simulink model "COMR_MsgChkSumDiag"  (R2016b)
settings: Solver=FixedStepDiscrete  StartTime=0.0  StopTime=10.0  FixedStep=0.01  RelTol=1e-3  EnableMultiTasking=on
undefined symbols (not defined in the file or in its folder): bin2dec, COMR_cntABM050ChkSumDiag_CW, COMR_cntOBCChkSumDiag_CW, COMR_cntVcu2A3ChkSumDiag_CW
libraries: simulink x34

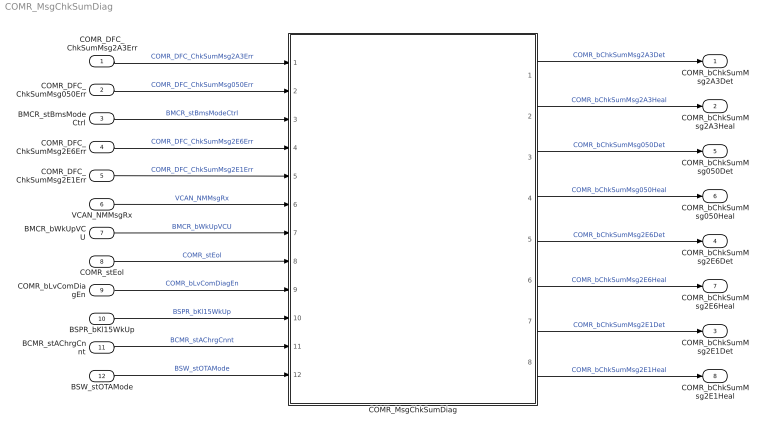
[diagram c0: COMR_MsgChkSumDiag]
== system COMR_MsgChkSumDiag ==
  COMR_DFC_ChkSumMsg2A3Err : Inport  OutDataTypeStr=boolean
  COMR_DFC_ChkSumMsg050Err : Inport  Port=2  OutDataTypeStr=boolean
  BMCR_stBmsModeCtrl : Inport  Port=3
  COMR_DFC_ChkSumMsg2E6Err : Inport  Port=4  OutDataTypeStr=boolean
  COMR_DFC_ChkSumMsg2E1Err : Inport  Port=5  OutDataTypeStr=boolean
  VCAN_NMMsgRx : Inport  Port=6  OutDataTypeStr=boolean
  BMCR_bWkUpVCU : Inport  Port=7  OutDataTypeStr=boolean
  COMR_stEol : Inport  Port=8  OutDataTypeStr=boolean
  COMR_bLvComDiagEn : Inport  Port=9  OutDataTypeStr=boolean
  BSPR_bKl15WkUp : Inport  Port=10
  BCMR_stAChrgCnnt : Inport  Port=11
  BSW_stOTAMode : Inport  Port=12  OutDataTypeStr=boolean
  COMR_MsgChkSumDiag : Subsystem
  COMR_bChkSumMsg2A3Det : Outport
  COMR_bChkSumMsg2A3Heal : Outport  Port=2
  COMR_bChkSumMsg2E1Det : Outport  Port=3
  COMR_bChkSumMsg2E6Det : Outport  Port=4
  COMR_bChkSumMsg050Det : Outport  Port=5
  COMR_bChkSumMsg050Heal : Outport  Port=6
  COMR_bChkSumMsg2E6Heal : Outport  Port=7
  COMR_bChkSumMsg2E1Heal : Outport  Port=8
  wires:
  COMR_DFC_ChkSumMsg2A3Err/1 -> COMR_MsgChkSumDiag/1(COMR_DFC_ChkSumMsg2A3Err)  "COMR_DFC_ChkSumMsg2A3Err"
  COMR_DFC_ChkSumMsg050Err/1 -> COMR_MsgChkSumDiag/2(COMR_DFC_ChkSumMsg050Err)  "COMR_DFC_ChkSumMsg050Err"
  COMR_DFC_ChkSumMsg2E6Err/1 -> COMR_MsgChkSumDiag/4(COMR_DFC_ChkSumMsg2E6Err)  "COMR_DFC_ChkSumMsg2E6Err"
  COMR_MsgChkSumDiag/1(COMR_bChkSumMsg2A3Det) -> COMR_bChkSumMsg2A3Det/1  "COMR_bChkSumMsg2A3Det"
  COMR_DFC_ChkSumMsg2E1Err/1 -> COMR_MsgChkSumDiag/5(COMR_DFC_ChkSumMsg2E1Err)  "COMR_DFC_ChkSumMsg2E1Err"
  COMR_MsgChkSumDiag/3(COMR_bChkSumMsg050Det) -> COMR_bChkSumMsg050Det/1  "COMR_bChkSumMsg050Det"
  COMR_MsgChkSumDiag/7(COMR_bChkSumMsg2E1Det) -> COMR_bChkSumMsg2E1Det/1  "COMR_bChkSumMsg2E1Det"
  COMR_MsgChkSumDiag/5(COMR_bChkSumMsg2E6Det) -> COMR_bChkSumMsg2E6Det/1  "COMR_bChkSumMsg2E6Det"
  BMCR_stBmsModeCtrl/1 -> COMR_MsgChkSumDiag/3(BMCR_stBmsModeCtrl)  "BMCR_stBmsModeCtrl"
  COMR_MsgChkSumDiag/2(COMR_bChkSumMsg2A3Heal) -> COMR_bChkSumMsg2A3Heal/1  "COMR_bChkSumMsg2A3Heal"
  COMR_MsgChkSumDiag/4(COMR_ChkSumMsg050Heal) -> COMR_bChkSumMsg050Heal/1  "COMR_bChkSumMsg050Heal"
  COMR_MsgChkSumDiag/6(COMR_bChkSumMsg2E6Heal) -> COMR_bChkSumMsg2E6Heal/1  "COMR_bChkSumMsg2E6Heal"
  COMR_MsgChkSumDiag/8(COMR_bChkSumMsg2E1Heal) -> COMR_bChkSumMsg2E1Heal/1  "COMR_bChkSumMsg2E1Heal"
  VCAN_NMMsgRx/1 -> COMR_MsgChkSumDiag/6(VCAN_NMMsgRx)  "VCAN_NMMsgRx"
  BMCR_bWkUpVCU/1 -> COMR_MsgChkSumDiag/7(BMCR_bWkUpVCU)  "BMCR_bWkUpVCU"
  COMR_stEol/1 -> COMR_MsgChkSumDiag/8(COMR_stEol)  "COMR_stEol"
  COMR_bLvComDiagEn/1 -> COMR_MsgChkSumDiag/9(COMR_bLvComDiagEn)  "COMR_bLvComDiagEn"
  BSPR_bKl15WkUp/1 -> COMR_MsgChkSumDiag/10(BSPR_bKl15WkUp)  "BSPR_bKl15WkUp"
  BCMR_stAChrgCnnt/1 -> COMR_MsgChkSumDiag/11(BCMR_stAChrgCnnt)  "BCMR_stAChrgCnnt"
  BSW_stOTAMode/1 -> COMR_MsgChkSumDiag/12(BSW_stOTAMode)  "BSW_stOTAMode"

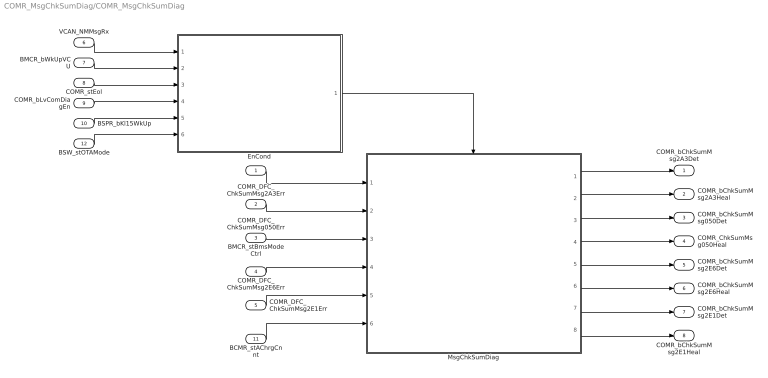
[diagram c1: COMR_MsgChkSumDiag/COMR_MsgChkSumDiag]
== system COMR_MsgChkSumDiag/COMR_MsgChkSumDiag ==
  COMR_DFC_ChkSumMsg2A3Err : Inport  OutDataTypeStr=boolean
  COMR_DFC_ChkSumMsg050Err : Inport  Port=2  OutDataTypeStr=boolean
  BMCR_stBmsModeCtrl : Inport  Port=3
  COMR_DFC_ChkSumMsg2E6Err : Inport  Port=4  OutDataTypeStr=boolean
  COMR_DFC_ChkSumMsg2E1Err : Inport  Port=5  OutDataTypeStr=boolean
  VCAN_NMMsgRx : Inport  Port=6  OutDataTypeStr=boolean
  BMCR_bWkUpVCU : Inport  Port=7  OutDataTypeStr=boolean
  COMR_stEol : Inport  Port=8  OutDataTypeStr=boolean
  COMR_bLvComDiagEn : Inport  Port=9  OutDataTypeStr=boolean
  BSPR_bKl15WkUp : Inport  Port=10
  BCMR_stAChrgCnnt : Inport  Port=11
  BSW_stOTAMode : Inport  Port=12  OutDataTypeStr=boolean
  EnCond : Subsystem
  MsgChkSumDiag : Subsystem
  COMR_bChkSumMsg2A3Det : Outport
  COMR_bChkSumMsg2A3Heal : Outport  Port=2
  COMR_bChkSumMsg050Det : Outport  Port=3
  COMR_ChkSumMsg050Heal : Outport  Port=4
  COMR_bChkSumMsg2E6Det : Outport  Port=5
  COMR_bChkSumMsg2E6Heal : Outport  Port=6
  COMR_bChkSumMsg2E1Det : Outport  Port=7
  COMR_bChkSumMsg2E1Heal : Outport  Port=8
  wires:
  COMR_DFC_ChkSumMsg2A3Err/1 -> MsgChkSumDiag/1(COMR_DFC_ChkSumMsg2A3Err)
  COMR_DFC_ChkSumMsg050Err/1 -> MsgChkSumDiag/2(COMR_DFC_ChkSumMsg050Err)
  BMCR_stBmsModeCtrl/1 -> MsgChkSumDiag/3(BMCR_stBmsModeCtrl)
  COMR_DFC_ChkSumMsg2E6Err/1 -> MsgChkSumDiag/4(COMR_DFC_ChkSumMsg2E6Err)
  COMR_DFC_ChkSumMsg2E1Err/1 -> MsgChkSumDiag/5(COMR_DFC_ChkSumMsg2E1Err)
  MsgChkSumDiag/1(COMR_bChkSumMsg2A3Det) -> COMR_bChkSumMsg2A3Det/1
  MsgChkSumDiag/2(COMR_bChkSumMsg2A3Heal) -> COMR_bChkSumMsg2A3Heal/1
  MsgChkSumDiag/3(COMR_bChkSumMsg050Det) -> COMR_bChkSumMsg050Det/1
  MsgChkSumDiag/4(COMR_ChkSumMsg050Heal) -> COMR_ChkSumMsg050Heal/1
  MsgChkSumDiag/5(COMR_bChkSumMsg2E6Det) -> COMR_bChkSumMsg2E6Det/1
  MsgChkSumDiag/6(COMR_bChkSumMsg2E6Heal) -> COMR_bChkSumMsg2E6Heal/1
  MsgChkSumDiag/7(COMR_bChkSumMsg2E1Det) -> COMR_bChkSumMsg2E1Det/1
  MsgChkSumDiag/8(COMR_bChkSumMsg2E1Heal) -> COMR_bChkSumMsg2E1Heal/1
  EnCond/1(COMR_bMsgChkSumDiagEn) -> MsgChkSumDiag/Enable
  VCAN_NMMsgRx/1 -> EnCond/1(VCAN_NMMsgRx)
  BMCR_bWkUpVCU/1 -> EnCond/2(BMCR_bWkUpVCU)
  COMR_stEol/1 -> EnCond/3(COMR_stEol)
  COMR_bLvComDiagEn/1 -> EnCond/4(COMR_bLvComDiagEn)
  BSPR_bKl15WkUp/1 -> EnCond/5(BSPR_bKl15WkUp)
  BCMR_stAChrgCnnt/1 -> MsgChkSumDiag/6(BCMR_stAChrgCnnt)
  BSW_stOTAMode/1 -> EnCond/6(BSW_stOTAMode)

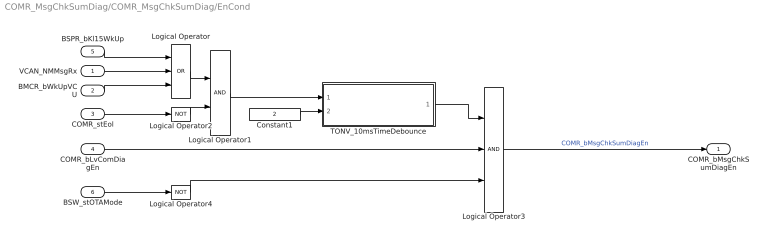
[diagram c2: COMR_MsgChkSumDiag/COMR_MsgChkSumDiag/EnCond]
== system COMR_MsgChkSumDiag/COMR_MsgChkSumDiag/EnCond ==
  VCAN_NMMsgRx : Inport  OutDataTypeStr=boolean
  BMCR_bWkUpVCU : Inport  Port=2  OutDataTypeStr=boolean
  COMR_stEol : Inport  Port=3  OutDataTypeStr=boolean
  COMR_bLvComDiagEn : Inport  Port=4  OutDataTypeStr=boolean
  BSPR_bKl15WkUp : Inport  Port=5
  BSW_stOTAMode : Inport  Port=6  OutDataTypeStr=boolean
  Constant1 : Constant  Value=2  OutDataTypeStr=single
  Logical Operator : Logic  Operator=OR  Inputs=3  AllPortsSameDT=off  OutDataTypeStr=boolean
  Logical Operator1 : Logic  AllPortsSameDT=off  OutDataTypeStr=boolean
  Logical Operator2 : Logic  Operator=NOT  AllPortsSameDT=off  OutDataTypeStr=boolean
  Logical Operator3 : Logic  Inputs=3  AllPortsSameDT=off  OutDataTypeStr=boolean
  Logical Operator4 : Logic  Operator=NOT  AllPortsSameDT=off  OutDataTypeStr=boolean
  TONV_10msTimeDebounce : Subsystem  TreatAsAtomicUnit=on  RTWFcnName=TONV_10msTimeDebounce  RTWFileName=SrvLib
  COMR_bMsgChkSumDiagEn : Outport
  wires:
  Logical Operator1/1 -> TONV_10msTimeDebounce/1(u)
  Constant1/1 -> TONV_10msTimeDebounce/2(T)
  Logical Operator3/1 -> COMR_bMsgChkSumDiagEn/1  "COMR_bMsgChkSumDiagEn"
  Logical Operator/1 -> Logical Operator1/1
  COMR_stEol/1 -> Logical Operator2/1
  Logical Operator2/1 -> Logical Operator1/2
  TONV_10msTimeDebounce/1(y) -> Logical Operator3/1
  COMR_bLvComDiagEn/1 -> Logical Operator3/2
  BMCR_bWkUpVCU/1 -> Logical Operator/3
  VCAN_NMMsgRx/1 -> Logical Operator/2
  BSPR_bKl15WkUp/1 -> Logical Operator/1
  BSW_stOTAMode/1 -> Logical Operator4/1
  Logical Operator4/1 -> Logical Operator3/3

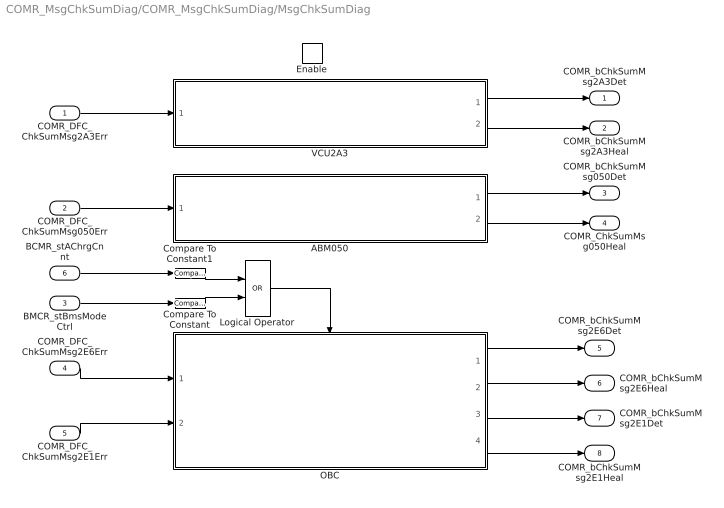
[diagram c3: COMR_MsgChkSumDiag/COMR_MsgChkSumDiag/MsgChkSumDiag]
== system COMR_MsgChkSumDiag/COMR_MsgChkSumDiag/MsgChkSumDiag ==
  COMR_DFC_ChkSumMsg2A3Err : Inport  OutDataTypeStr=boolean
  COMR_DFC_ChkSumMsg050Err : Inport  Port=2  OutDataTypeStr=boolean
  BMCR_stBmsModeCtrl : Inport  Port=3
  COMR_DFC_ChkSumMsg2E6Err : Inport  Port=4  OutDataTypeStr=boolean
  COMR_DFC_ChkSumMsg2E1Err : Inport  Port=5  OutDataTypeStr=boolean
  BCMR_stAChrgCnnt : Inport  Port=6
  Enable : EnablePort  StatesWhenEnabling=reset
  ABM050 : Subsystem
  Compare To Constant : simulink/Logic and Bit Operations/Compare To Constant  relop===  const=6  OutDataTypeStr=boolean
  Compare To Constant1 : simulink/Logic and Bit Operations/Compare To Constant  relop===  const=1  OutDataTypeStr=boolean
  Logical Operator : Logic  Operator=OR  AllPortsSameDT=off  OutDataTypeStr=boolean
  OBC : Subsystem
  VCU2A3 : Subsystem
  COMR_bChkSumMsg2A3Det : Outport
  COMR_bChkSumMsg2A3Heal : Outport  Port=2
  COMR_bChkSumMsg050Det : Outport  Port=3
  COMR_ChkSumMsg050Heal : Outport  Port=4
  COMR_bChkSumMsg2E6Det : Outport  Port=5  InitialOutput=[0]
  COMR_bChkSumMsg2E6Heal : Outport  Port=6  InitialOutput=[0]
  COMR_bChkSumMsg2E1Det : Outport  Port=7  InitialOutput=[0]
  COMR_bChkSumMsg2E1Heal : Outport  Port=8  InitialOutput=[0]
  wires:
  OBC/4(COMR_bChkSumMsg2E1Heal) -> COMR_bChkSumMsg2E1Heal/1
  ABM050/2(COMR_bChkSumMsg050Heal) -> COMR_ChkSumMsg050Heal/1
  COMR_DFC_ChkSumMsg050Err/1 -> ABM050/1(COMR_DFC_ChkSumMsg050Err)
  OBC/2(COMR_bChkSumMsg2E6Heal) -> COMR_bChkSumMsg2E6Heal/1
  ABM050/1(COMR_bChkSumMsg050Det) -> COMR_bChkSumMsg050Det/1
  VCU2A3/2(COMR_bChkSumMsg2A3Heal) -> COMR_bChkSumMsg2A3Heal/1
  OBC/3(COMR_bChkSumMsg2E1Det) -> COMR_bChkSumMsg2E1Det/1
  COMR_DFC_ChkSumMsg2E6Err/1 -> OBC/1(BSWOBC2E0CheckSum)
  BMCR_stBmsModeCtrl/1 -> Compare To Constant/1
  COMR_DFC_ChkSumMsg2E1Err/1 -> OBC/2(BSWOBC2E1CheckSum)
  VCU2A3/1(COMR_bChkSumMsg2A3Det) -> COMR_bChkSumMsg2A3Det/1
  COMR_DFC_ChkSumMsg2A3Err/1 -> VCU2A3/1(COMR_DFC_ChkSumMsg2A3Err)
  OBC/1(COMR_bChkSumMsg2E6Det) -> COMR_bChkSumMsg2E6Det/1
  BCMR_stAChrgCnnt/1 -> Compare To Constant1/1
  Compare To Constant1/1 -> Logical Operator/1
  Compare To Constant/1 -> Logical Operator/2
  Logical Operator/1 -> OBC/Enable

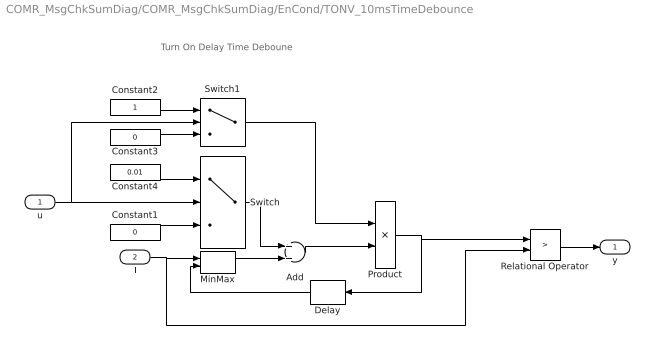
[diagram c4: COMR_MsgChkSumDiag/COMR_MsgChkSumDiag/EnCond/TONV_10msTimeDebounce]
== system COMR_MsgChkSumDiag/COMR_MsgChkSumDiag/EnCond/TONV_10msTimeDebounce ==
  note: Turn On Delay Time Deboune
  u : Inport
  T : Inport  Port=2
  Add : Sum
  Constant1 : Constant  Value=0  OutDataTypeStr=single
  Constant2 : Constant  OutDataTypeStr=uint8
  Constant3 : Constant  Value=0  OutDataTypeStr=uint8
  Constant4 : Constant  Value=0.01  OutDataTypeStr=single
  Delay : Delay  DelayLength=1  InitialCondition=0
  MinMax : MinMax  Inputs=2
  Product : Product  OutMin=[0]  OutMax=[65535]  OutDataTypeStr=single
  Relational Operator : RelationalOperator  Operator=>  OutDataTypeStr=boolean  RndMeth=Simplest
  Switch : Switch  Criteria=u2 ~= 0
  Switch1 : Switch  Criteria=u2 ~= 0
  y : Outport
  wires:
  MinMax/1 -> Add/2
  T/1 -> Relational Operator/2, MinMax/1
  Relational Operator/1 -> y/1
  Delay/1 -> MinMax/2
  Switch/1 -> Add/1
  Product/1 -> Delay/1, Relational Operator/1
  Add/1 -> Product/2
  Constant1/1 -> Switch/3
  Constant4/1 -> Switch/1
  u/1 -> Switch/2, Switch1/2
  Constant2/1 -> Switch1/1
  Constant3/1 -> Switch1/3
  Switch1/1 -> Product/1

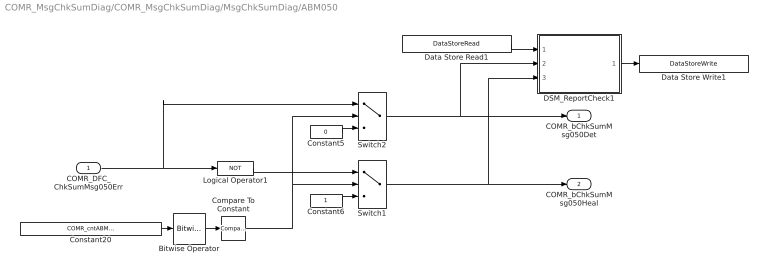
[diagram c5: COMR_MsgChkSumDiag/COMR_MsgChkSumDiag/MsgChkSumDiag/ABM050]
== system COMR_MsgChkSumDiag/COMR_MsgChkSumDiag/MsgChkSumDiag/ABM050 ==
  COMR_DFC_ChkSumMsg050Err : Inport  OutDataTypeStr=boolean
  Bitwise Operator : simulink/Logic and Bit Operations/Bitwise Operator  logicop=AND  UseBitMask=on  BitMask=bin2dec('00010000')  BitMaskRealWorld=Stored Integer
  Compare To Constant : simulink/Logic and Bit Operations/Compare To Constant  relop===  const=16  OutDataTypeStr=boolean
  Constant20 : Constant  Value=COMR_cntABM050ChkSumDiag_CW
  Constant5 : Constant  Value=0  OutDataTypeStr=boolean
  Constant6 : Constant  OutDataTypeStr=boolean
  DSM_ReportCheck1 : Subsystem  TreatAsAtomicUnit=on  RTWFcnName=DSM_ReportCheck  RTWFileName=SrvLib
  Data Store Read1 : DataStoreRead  DataStoreName=DFC_ChkSumMsg050Err
  Data Store Write1 : DataStoreWrite  DataStoreName=DFC_ChkSumMsg050Err
  Logical Operator1 : Logic  Operator=NOT  AllPortsSameDT=off  OutDataTypeStr=boolean
  Switch1 : Switch  Criteria=u2 > Threshold
  Switch2 : Switch  Criteria=u2 > Threshold
  COMR_bChkSumMsg050Det : Outport
  COMR_bChkSumMsg050Heal : Outport  Port=2
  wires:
  Constant6/1 -> Switch1/3
  Constant5/1 -> Switch2/3
  Bitwise Operator/1 -> Compare To Constant/1
  Constant20/1 -> Bitwise Operator/1
  Compare To Constant/1 -> Switch2/2, Switch1/2
  Switch2/1 -> DSM_ReportCheck1/2(Err), COMR_bChkSumMsg050Det/1
  DSM_ReportCheck1/1(Dfc_id) -> Data Store Write1/1
  Switch1/1 -> DSM_ReportCheck1/3(Heal), COMR_bChkSumMsg050Heal/1
  Data Store Read1/1 -> DSM_ReportCheck1/1(Dfc_id_nv)
  COMR_DFC_ChkSumMsg050Err/1 -> Switch2/1, Logical Operator1/1
  Logical Operator1/1 -> Switch1/1

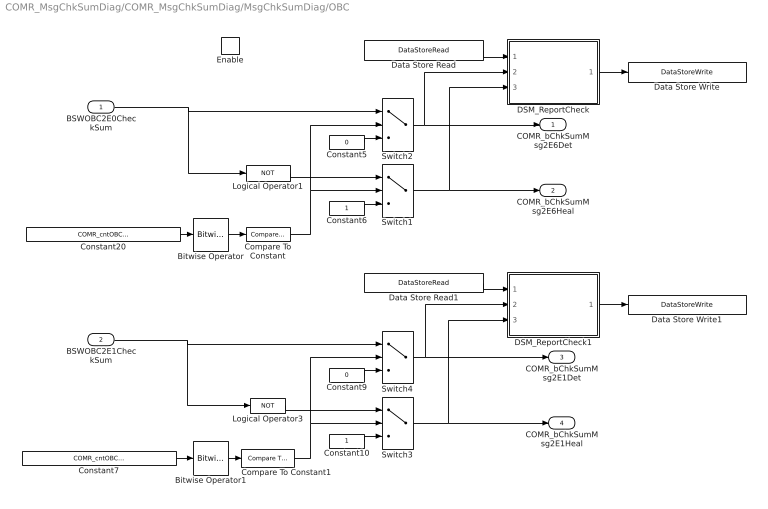
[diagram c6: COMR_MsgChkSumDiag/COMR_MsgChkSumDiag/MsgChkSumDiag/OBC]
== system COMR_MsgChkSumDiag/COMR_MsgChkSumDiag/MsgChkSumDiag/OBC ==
  BSWOBC2E0CheckSum : Inport  OutDataTypeStr=boolean
  BSWOBC2E1CheckSum : Inport  Port=2  OutDataTypeStr=boolean
  Enable : EnablePort  StatesWhenEnabling=reset
  Bitwise Operator : simulink/Logic and Bit Operations/Bitwise Operator  logicop=AND  UseBitMask=on  BitMask=bin2dec('00010000')  BitMaskRealWorld=Stored Integer
  Bitwise Operator1 : simulink/Logic and Bit Operations/Bitwise Operator  logicop=AND  UseBitMask=on  BitMask=bin2dec('00010000')  BitMaskRealWorld=Stored Integer
  Compare To Constant : simulink/Logic and Bit Operations/Compare To Constant  relop===  const=16  OutDataTypeStr=boolean
  Compare To Constant1 : simulink/Logic and Bit Operations/Compare To Constant  relop===  const=16  OutDataTypeStr=boolean
  Constant10 : Constant  OutDataTypeStr=boolean
  Constant20 : Constant  Value=COMR_cntOBCChkSumDiag_CW
  Constant5 : Constant  Value=0  OutDataTypeStr=boolean
  Constant6 : Constant  OutDataTypeStr=boolean
  Constant7 : Constant  Value=COMR_cntOBCChkSumDiag_CW
  Constant9 : Constant  Value=0  OutDataTypeStr=boolean
  DSM_ReportCheck : Subsystem  TreatAsAtomicUnit=on  RTWFcnName=DSM_ReportCheck  RTWFileName=SrvLib
  DSM_ReportCheck1 : Subsystem  TreatAsAtomicUnit=on  RTWFcnName=DSM_ReportCheck  RTWFileName=SrvLib
  Data Store Read : DataStoreRead  DataStoreName=DFC_ChkSumMsg2E0Err
  Data Store Read1 : DataStoreRead  DataStoreName=DFC_ChkSumMsg2E1Err
  Data Store Write : DataStoreWrite  DataStoreName=DFC_ChkSumMsg2E0Err
  Data Store Write1 : DataStoreWrite  DataStoreName=DFC_ChkSumMsg2E1Err
  Logical Operator1 : Logic  Operator=NOT  AllPortsSameDT=off  OutDataTypeStr=boolean
  Logical Operator3 : Logic  Operator=NOT  AllPortsSameDT=off  OutDataTypeStr=boolean
  Switch{1..4} (4 alike) : Switch  Criteria=u2 > Threshold
  COMR_bChkSumMsg2E6Det : Outport
  COMR_bChkSumMsg2E6Heal : Outport  Port=2
  COMR_bChkSumMsg2E1Det : Outport  Port=3
  COMR_bChkSumMsg2E1Heal : Outport  Port=4
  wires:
  Constant6/1 -> Switch1/3
  Constant5/1 -> Switch2/3
  Bitwise Operator/1 -> Compare To Constant/1
  Constant20/1 -> Bitwise Operator/1
  Compare To Constant/1 -> Switch2/2, Switch1/2
  Data Store Read/1 -> DSM_ReportCheck/1(Dfc_id_nv)
  DSM_ReportCheck/1(Dfc_id) -> Data Store Write/1
  Switch1/1 -> COMR_bChkSumMsg2E6Heal/1, DSM_ReportCheck/3(Heal)
  Switch2/1 -> DSM_ReportCheck/2(Err), COMR_bChkSumMsg2E6Det/1
  Constant10/1 -> Switch3/3
  Constant9/1 -> Switch4/3
  Bitwise Operator1/1 -> Compare To Constant1/1
  Constant7/1 -> Bitwise Operator1/1
  Compare To Constant1/1 -> Switch4/2, Switch3/2
  DSM_ReportCheck1/1(Dfc_id) -> Data Store Write1/1
  Switch3/1 -> COMR_bChkSumMsg2E1Heal/1, DSM_ReportCheck1/3(Heal)
  Switch4/1 -> COMR_bChkSumMsg2E1Det/1, DSM_ReportCheck1/2(Err)
  Data Store Read1/1 -> DSM_ReportCheck1/1(Dfc_id_nv)
  BSWOBC2E0CheckSum/1 -> Logical Operator1/1, Switch2/1
  Logical Operator1/1 -> Switch1/1
  Logical Operator3/1 -> Switch3/1
  BSWOBC2E1CheckSum/1 -> Logical Operator3/1, Switch4/1

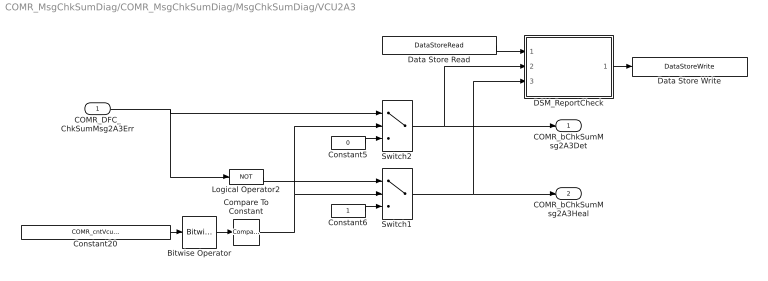
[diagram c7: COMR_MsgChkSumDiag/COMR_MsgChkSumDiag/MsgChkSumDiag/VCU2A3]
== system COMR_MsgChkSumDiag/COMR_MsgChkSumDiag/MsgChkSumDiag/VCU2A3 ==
  COMR_DFC_ChkSumMsg2A3Err : Inport  OutDataTypeStr=boolean
  Bitwise Operator : simulink/Logic and Bit Operations/Bitwise Operator  logicop=AND  UseBitMask=on  BitMask=bin2dec('00010000')  BitMaskRealWorld=Stored Integer
  Compare To Constant : simulink/Logic and Bit Operations/Compare To Constant  relop===  const=16  OutDataTypeStr=boolean
  Constant20 : Constant  Value=COMR_cntVcu2A3ChkSumDiag_CW
  Constant5 : Constant  Value=0  OutDataTypeStr=boolean
  Constant6 : Constant  OutDataTypeStr=boolean
  DSM_ReportCheck : Subsystem  TreatAsAtomicUnit=on  RTWFcnName=DSM_ReportCheck  RTWFileName=SrvLib
  Data Store Read : DataStoreRead  DataStoreName=DFC_ChkSumMsg2A3Err
  Data Store Write : DataStoreWrite  DataStoreName=DFC_ChkSumMsg2A3Err
  Logical Operator2 : Logic  Operator=NOT  AllPortsSameDT=off  OutDataTypeStr=boolean
  Switch1 : Switch  Criteria=u2 > Threshold
  Switch2 : Switch  Criteria=u2 > Threshold
  COMR_bChkSumMsg2A3Det : Outport
  COMR_bChkSumMsg2A3Heal : Outport  Port=2
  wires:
  COMR_DFC_ChkSumMsg2A3Err/1 -> Switch2/1, Logical Operator2/1
  Constant20/1 -> Bitwise Operator/1
  Compare To Constant/1 -> Switch1/2, Switch2/2
  Constant5/1 -> Switch2/3
  Bitwise Operator/1 -> Compare To Constant/1
  Constant6/1 -> Switch1/3
  Switch2/1 -> DSM_ReportCheck/2(Err), COMR_bChkSumMsg2A3Det/1
  DSM_ReportCheck/1(Dfc_id) -> Data Store Write/1
  Switch1/1 -> DSM_ReportCheck/3(Heal), COMR_bChkSumMsg2A3Heal/1
  Data Store Read/1 -> DSM_ReportCheck/1(Dfc_id_nv)
  Logical Operator2/1 -> Switch1/1

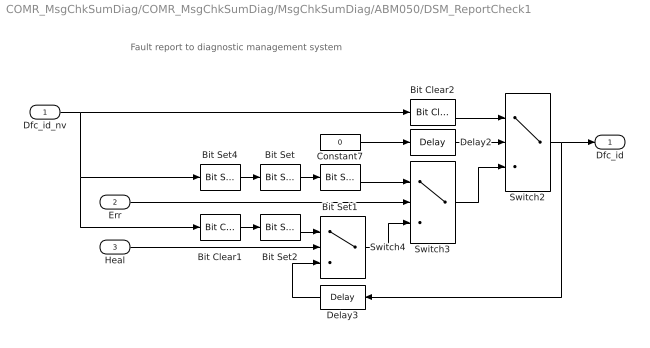
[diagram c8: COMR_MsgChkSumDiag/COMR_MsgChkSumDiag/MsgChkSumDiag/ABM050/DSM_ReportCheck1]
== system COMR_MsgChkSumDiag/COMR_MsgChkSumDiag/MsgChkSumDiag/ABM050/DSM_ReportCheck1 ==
  note: Fault report to diagnostic management system
  Dfc_id_nv : Inport  OutDataTypeStr=uint8
  Err : Inport  Port=2
  Heal : Inport  Port=3
  Bit Clear1 : simulink/Logic and Bit Operations/Bit Clear  iBit=4
  Bit Clear2 : simulink/Logic and Bit Operations/Bit Clear  iBit=3
  Bit Set : simulink/Logic and Bit Operations/Bit Set  iBit=4
  Bit Set1 : simulink/Logic and Bit Operations/Bit Set  iBit=3
  Bit Set2 : simulink/Logic and Bit Operations/Bit Set  iBit=3
  Bit Set4 : simulink/Logic and Bit Operations/Bit Set  iBit=7
  Constant7 : Constant  Value=0  OutDataTypeStr=boolean
  Delay2 : Delay  DelayLength=1  InitialCondition=1
  Delay3 : Delay  DelayLength=1  InitialCondition=0
  Switch2 : Switch  Criteria=u2 ~= 0
  Switch3 : Switch  Criteria=u2 ~= 0
  Switch4 : Switch  Criteria=u2 ~= 0
  Dfc_id : Outport  OutDataTypeStr=uint8
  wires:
  Dfc_id_nv/1 -> Bit Clear2/1, Bit Set4/1, Bit Clear1/1
  Bit Set4/1 -> Bit Set/1
  Constant7/1 -> Delay2/1
  Delay2/1 -> Switch2/2
  Switch3/1 -> Switch2/3
  Bit Clear2/1 -> Switch2/1
  Switch2/1 -> Delay3/1, Dfc_id/1
  Bit Set1/1 -> Switch3/1
  Bit Set/1 -> Bit Set1/1
  Switch4/1 -> Switch3/3
  Err/1 -> Switch3/2
  Bit Set2/1 -> Switch4/1
  Bit Clear1/1 -> Bit Set2/1
  Delay3/1 -> Switch4/3
  Heal/1 -> Switch4/2

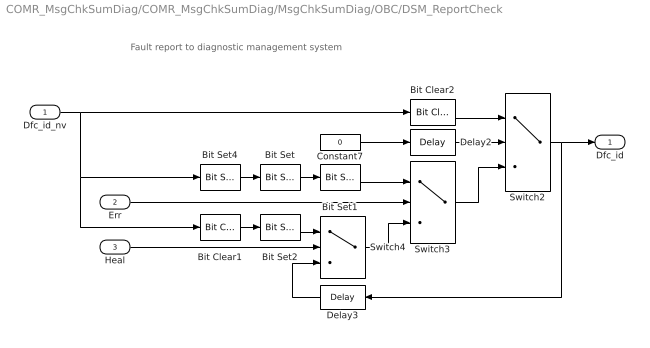
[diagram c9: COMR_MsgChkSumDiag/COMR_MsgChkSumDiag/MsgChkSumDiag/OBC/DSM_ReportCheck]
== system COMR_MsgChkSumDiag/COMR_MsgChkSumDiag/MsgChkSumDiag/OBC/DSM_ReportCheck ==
  note: Fault report to diagnostic management system
  Dfc_id_nv : Inport  OutDataTypeStr=uint8
  Err : Inport  Port=2
  Heal : Inport  Port=3
  Bit Clear1 : simulink/Logic and Bit Operations/Bit Clear  iBit=4
  Bit Clear2 : simulink/Logic and Bit Operations/Bit Clear  iBit=3
  Bit Set : simulink/Logic and Bit Operations/Bit Set  iBit=4
  Bit Set1 : simulink/Logic and Bit Operations/Bit Set  iBit=3
  Bit Set2 : simulink/Logic and Bit Operations/Bit Set  iBit=3
  Bit Set4 : simulink/Logic and Bit Operations/Bit Set  iBit=7
  Constant7 : Constant  Value=0  OutDataTypeStr=boolean
  Delay2 : Delay  DelayLength=1  InitialCondition=1
  Delay3 : Delay  DelayLength=1  InitialCondition=0
  Switch2 : Switch  Criteria=u2 ~= 0
  Switch3 : Switch  Criteria=u2 ~= 0
  Switch4 : Switch  Criteria=u2 ~= 0
  Dfc_id : Outport  OutDataTypeStr=uint8
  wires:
  Dfc_id_nv/1 -> Bit Clear2/1, Bit Set4/1, Bit Clear1/1
  Bit Set4/1 -> Bit Set/1
  Constant7/1 -> Delay2/1
  Delay2/1 -> Switch2/2
  Switch3/1 -> Switch2/3
  Bit Clear2/1 -> Switch2/1
  Switch2/1 -> Delay3/1, Dfc_id/1
  Bit Set1/1 -> Switch3/1
  Bit Set/1 -> Bit Set1/1
  Switch4/1 -> Switch3/3
  Err/1 -> Switch3/2
  Bit Set2/1 -> Switch4/1
  Bit Clear1/1 -> Bit Set2/1
  Delay3/1 -> Switch4/3
  Heal/1 -> Switch4/2

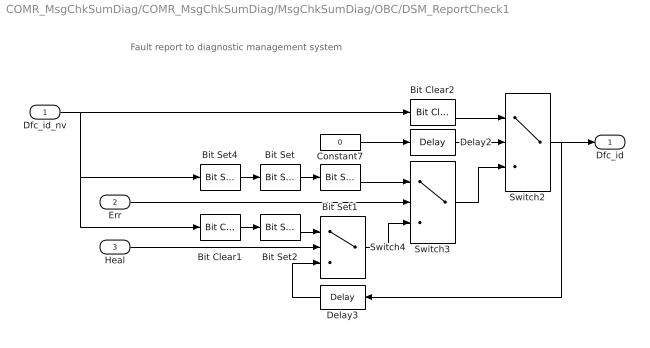
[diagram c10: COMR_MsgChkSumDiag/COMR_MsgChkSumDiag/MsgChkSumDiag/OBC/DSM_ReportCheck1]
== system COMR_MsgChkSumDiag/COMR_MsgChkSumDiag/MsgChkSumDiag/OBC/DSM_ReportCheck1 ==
  note: Fault report to diagnostic management system
  Dfc_id_nv : Inport  OutDataTypeStr=uint8
  Err : Inport  Port=2
  Heal : Inport  Port=3
  Bit Clear1 : simulink/Logic and Bit Operations/Bit Clear  iBit=4
  Bit Clear2 : simulink/Logic and Bit Operations/Bit Clear  iBit=3
  Bit Set : simulink/Logic and Bit Operations/Bit Set  iBit=4
  Bit Set1 : simulink/Logic and Bit Operations/Bit Set  iBit=3
  Bit Set2 : simulink/Logic and Bit Operations/Bit Set  iBit=3
  Bit Set4 : simulink/Logic and Bit Operations/Bit Set  iBit=7
  Constant7 : Constant  Value=0  OutDataTypeStr=boolean
  Delay2 : Delay  DelayLength=1  InitialCondition=1
  Delay3 : Delay  DelayLength=1  InitialCondition=0
  Switch2 : Switch  Criteria=u2 ~= 0
  Switch3 : Switch  Criteria=u2 ~= 0
  Switch4 : Switch  Criteria=u2 ~= 0
  Dfc_id : Outport  OutDataTypeStr=uint8
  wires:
  Dfc_id_nv/1 -> Bit Clear2/1, Bit Set4/1, Bit Clear1/1
  Bit Set4/1 -> Bit Set/1
  Constant7/1 -> Delay2/1
  Delay2/1 -> Switch2/2
  Switch3/1 -> Switch2/3
  Bit Clear2/1 -> Switch2/1
  Switch2/1 -> Delay3/1, Dfc_id/1
  Bit Set1/1 -> Switch3/1
  Bit Set/1 -> Bit Set1/1
  Switch4/1 -> Switch3/3
  Err/1 -> Switch3/2
  Bit Set2/1 -> Switch4/1
  Bit Clear1/1 -> Bit Set2/1
  Delay3/1 -> Switch4/3
  Heal/1 -> Switch4/2

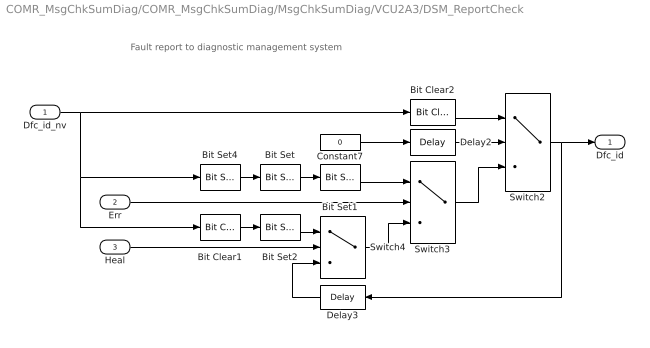
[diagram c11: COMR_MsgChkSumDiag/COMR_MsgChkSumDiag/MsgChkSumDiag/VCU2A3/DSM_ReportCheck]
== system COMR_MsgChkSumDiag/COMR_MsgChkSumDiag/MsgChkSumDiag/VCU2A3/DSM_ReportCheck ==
  note: Fault report to diagnostic management system
  Dfc_id_nv : Inport  OutDataTypeStr=uint8
  Err : Inport  Port=2
  Heal : Inport  Port=3
  Bit Clear1 : simulink/Logic and Bit Operations/Bit Clear  iBit=4
  Bit Clear2 : simulink/Logic and Bit Operations/Bit Clear  iBit=3
  Bit Set : simulink/Logic and Bit Operations/Bit Set  iBit=4
  Bit Set1 : simulink/Logic and Bit Operations/Bit Set  iBit=3
  Bit Set2 : simulink/Logic and Bit Operations/Bit Set  iBit=3
  Bit Set4 : simulink/Logic and Bit Operations/Bit Set  iBit=7
  Constant7 : Constant  Value=0  OutDataTypeStr=boolean
  Delay2 : Delay  DelayLength=1  InitialCondition=1
  Delay3 : Delay  DelayLength=1  InitialCondition=0
  Switch2 : Switch  Criteria=u2 ~= 0
  Switch3 : Switch  Criteria=u2 ~= 0
  Switch4 : Switch  Criteria=u2 ~= 0
  Dfc_id : Outport  OutDataTypeStr=uint8
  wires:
  Dfc_id_nv/1 -> Bit Clear2/1, Bit Set4/1, Bit Clear1/1
  Bit Set4/1 -> Bit Set/1
  Constant7/1 -> Delay2/1
  Delay2/1 -> Switch2/2
  Switch3/1 -> Switch2/3
  Bit Clear2/1 -> Switch2/1
  Switch2/1 -> Delay3/1, Dfc_id/1
  Bit Set1/1 -> Switch3/1
  Bit Set/1 -> Bit Set1/1
  Switch4/1 -> Switch3/3
  Err/1 -> Switch3/2
  Bit Set2/1 -> Switch4/1
  Bit Clear1/1 -> Bit Set2/1
  Delay3/1 -> Switch4/3
  Heal/1 -> Switch4/2
